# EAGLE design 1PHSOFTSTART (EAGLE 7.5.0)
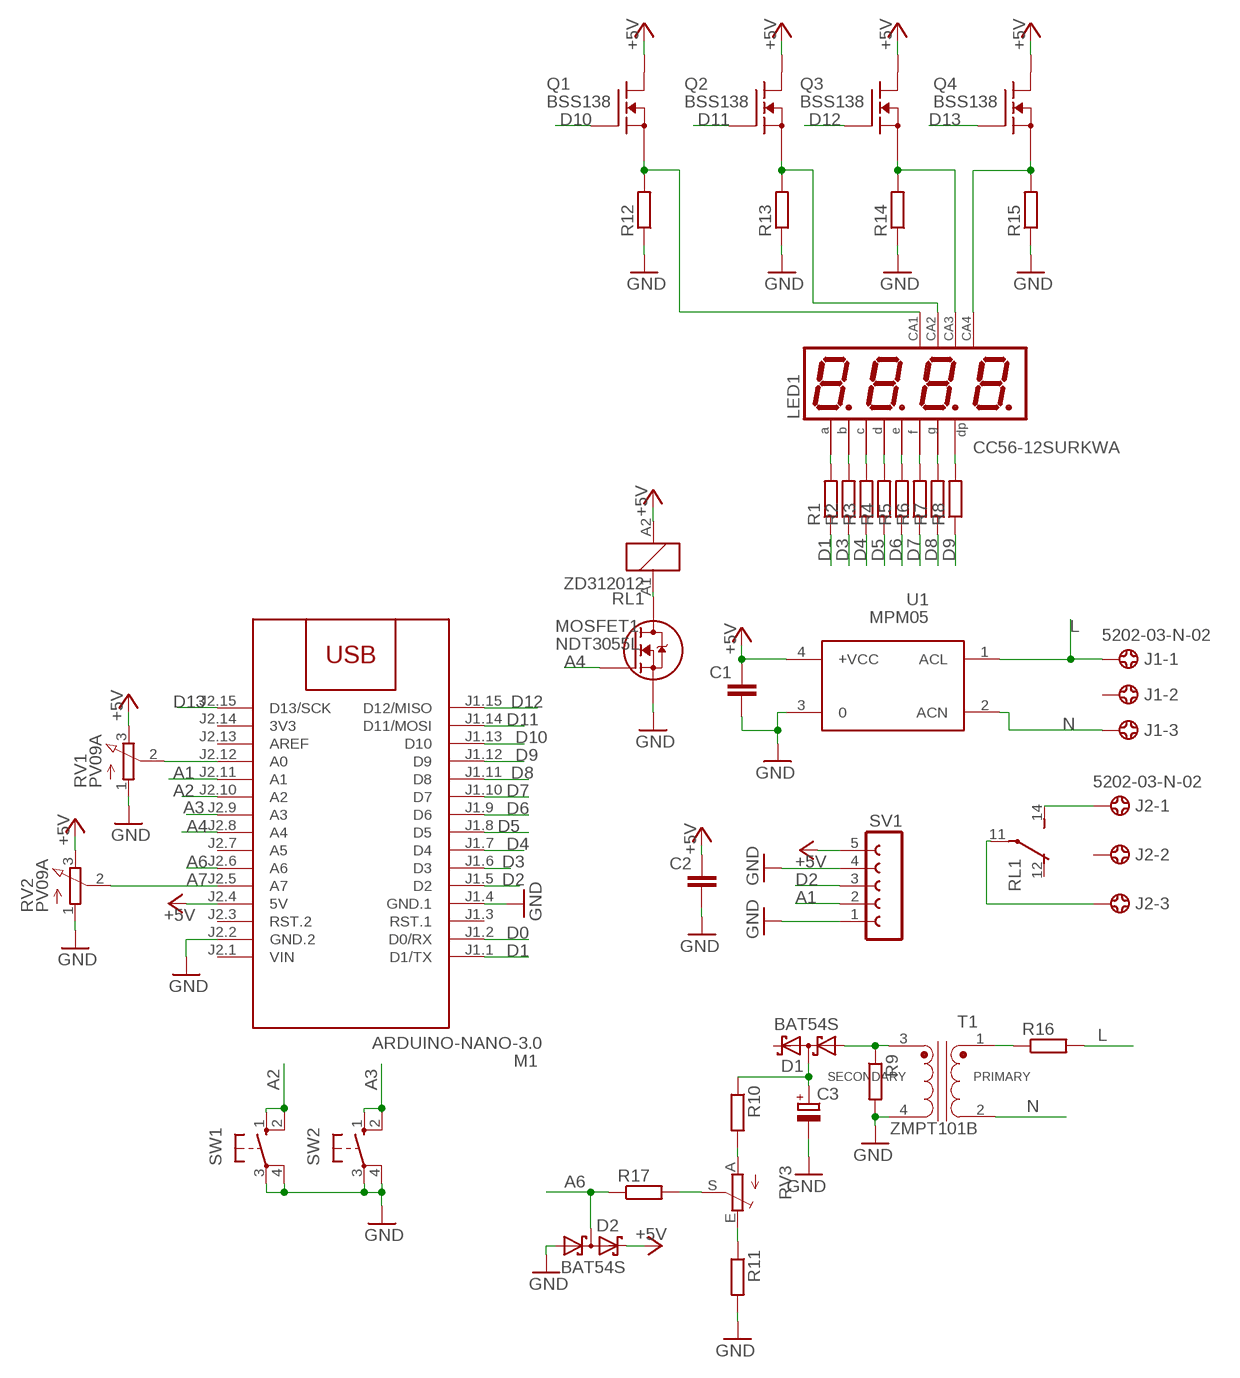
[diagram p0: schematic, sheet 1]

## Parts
C1  C-EUC1206  [C1206]
C2  C-EUC1206  [C1206]
C3  CPOL-EUSMCD  [SMC_D]
D1  BAT54S  [SOT23]
D2  BAT54S  [SOT23]
J1  5202-03-N-02  [5202-03-N-02]
J2  5202-03-N-02  [5202-03-N-02]
LED1  CC56-12SURKWA  CA56-12SURKWA  [CA56-12SURKWA]
M1  ARDUINO-NANO-3.0  [ARDUINO-NANO-3.0]
MOSFET1  NDT3055L  [SOT223-4]
Q1  BSS138  [SOT23]
Q2  BSS138  [SOT23]
Q3  BSS138  [SOT23]
Q4  BSS138  [SOT23]
R1  R-EU_R1206  [R1206]
R2  R-EU_R1206  [R1206]
R3  R-EU_R1206  [R1206]
R4  R-EU_R1206  [R1206]
R5  R-EU_R1206  [R1206]
R6  R-EU_R1206  [R1206]
R7  R-EU_R1206  [R1206]
R8  R-EU_R1206  [R1206]
R9  R-EU_R1206  [R1206]
R10  R-EU_R1206  [R1206]
R11  R-EU_R1206  [R1206]
R12  R-EU_R1206  [R1206]
R13  R-EU_R1206  [R1206]
R14  R-EU_R1206  [R1206]
R15  R-EU_R1206  [R1206]
R16  R-EU_R1206  [R1206]
R17  R-EU_R1206  [R1206]
RL1  ZD312012  [ZD1]
RV1  PV09A  [PTV09]
RV2  PV09A  [PTV09]
RV3  TRIM_EU-B25P  [B25P]
SV1  FE05-1  [FE05-1]
SW1  10-XX  [B3F-10XX]
SW2  10-XX  [B3F-10XX]
T1  ZMPT101B  [XFMR_ZMPT101B]
U1  MPM05  [MPM05]

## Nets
+5V: C1.1 C2.1 D2.2(C2) M1.J2.4(5V) Q1.2(D) Q2.2(D) Q3.2(D) Q4.2(D) RL1.A2 RV1.3(E) RV2.3(E) SV1.5 U1.4(+VCC)
A1: M1.J2.11(A1) SV1.2
A2: M1.J2.10(A2) SW1.1(S) SW1.2(S1)
A3: M1.J2.9(A3) SW2.1(S) SW2.2(S1)
A4: M1.J2.8(A4) MOSFET1.1(G)
A6: D2.3(C1A2) M1.J2.6(A6) R17.1
A7: M1.J2.5(A7) RV2.2(S)
D0: M1.J1.2(D0/RX)
D1: M1.J1.1(D1/TX) R1.1
D2: M1.J1.5(D2) SV1.3
D3: M1.J1.6(D3) R2.1
D4: M1.J1.7(D4) R3.1
D5: M1.J1.8(D5) R4.1
D6: M1.J1.9(D6) R5.1
D7: M1.J1.10(D7) R6.1
D8: M1.J1.11(D8) R7.1
D9: M1.J1.12(D9) R8.1
D10: M1.J1.13(D10) Q1.3(G)
D11: M1.J1.14(D11/MOSI) Q2.3(G)
D12: M1.J1.15(D12/MISO) Q3.3(G)
D13: M1.J2.15(D13/SCK) Q4.3(G)
GND: C1.2 C2.2 C3.- D2.1(A1) M1.J1.4(GND.1) M1.J2.2(GND.2) MOSFET1.3(S) R9.2 R11.2 R12.1 R13.1 R14.1 R15.1 RV1.1(A) RV2.1(A) SV1.1 SV1.4 SW1.3(P) SW1.4(P1) SW2.3(P) SW2.4(P1) T1.4 U1.3
L: J1.1 R16.2 U1.1(ACL)
N: J1.3 T1.2 U1.2(ACN)
N$1: M1.J2.12(A0) RV1.2(S)
N$2: J2.1 RL1.14(2:S)
N$3: J2.3 RL1.11(2:P)
N$4: D1.1(A1) R9.1 T1.3
N$5: R16.1 T1.1
N$6: C3.+ D1.3(C1A2) R10.1
N$7: R10.2 RV3.A
N$8: R17.2 RV3.S
N$9: R11.1 RV3.E
N$10: LED1.11(A) R1.2
N$11: LED1.7(B) R2.2
N$12: MOSFET1.2(D) MOSFET1.4(D) RL1.A1
N$15: LED1.4(C) R3.2
N$16: LED1.2(D) R4.2
N$17: LED1.1(E) R5.2
N$18: LED1.10(F) R6.2
N$19: LED1.5(G) R7.2
N$20: LED1.3(DP) R8.2
N$21: LED1.12(CA) Q1.1(S) R12.2
N$22: LED1.9(CA) Q2.1(S) R13.2
N$23: LED1.8(CA) Q3.1(S) R14.2
N$24: LED1.6(CA4) Q4.1(S) R15.2
Unconnected: D1.2(C2) J1.2 J2.2 M1.J1.3(RST.1) M1.J2.3(RST.2) M1.J2.7(A5) M1.J2.13(AREF) RL1.12(2:O)

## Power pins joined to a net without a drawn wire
3V3: M1.J2.14(3V3)
VIN: M1.J2.1(VIN)

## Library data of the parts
C1 C2 = rcl:C-EU: CAPACITOR, European symbol
C3 = rcl:CPOL-EU: POLARIZED CAPACITOR, European symbol
D1 D2 = diode:BAT54S: Schottky Diodes Pin connection corrected 2011-05-04 Source: Fairchild .. BAT54.pdf
J1 J2 = con-ebyelectro:5202-03-N-02: Barrier Blocks Sreies 5202 Source: http://www.ebyelectro.com/PDF/5202-XX-N-02.pdf; OC_FARNELL: unknown; OC_NEWARK: unknown
LED1 = display-kingbright:CA56-12SURKWA
M1 = diy-modules:ARDUINO-NANO-3.0: Arduino Nano 3.0 and compatible devices More details available here: https://www.arduino.cc/en/Main/ArduinoBoardNano Click here to find device on ebay.com
MOSFET1 = NDT3055L:NDT3055L: Trans MOSFET N-CH 60V 4A 4-Pin(3+Tab) SOT-223 Trans MOSFET N-CH 60V 4A 4-Pin(3+Tab) SOT-223 Check availability; AVAILABILITY: In Stock; CHECK_PRICES: https://www.snapeda.com/parts/NDT3055L/Onsemi/view-part/?ref=eda; DESCRIPTION: Trans MOSFET N-CH 60V 4A 4-Pin(3+Tab) SOT-223 Trans MOSFET N-CH 60V 4A 4-Pin(3+Tab) SOT-223; MF: ON; MP: NDT3055L; PACKAGE: SOT-223-4 Fairchild Semiconductor; PRICE: None; SNAPEDA_LINK: https://www.snapeda.com/parts/NDT3055L/Onsemi/view-part/?ref=snap
Q1-Q4 = transistor-fet:BSS138
R1-R17 = rcl:R-EU_: RESISTOR, European symbol
RL1 = relay:ZD?1*: Power Relay SCHRACK 1 pole 30 A Source: http://www.schrack.com/.. 5848.pdf; OC_FARNELL: unknown; OC_NEWARK: unknown
RV1 RV2 = pot:PV09A
RV3 = pot:TRIM_EU-: POTENTIOMETER
SV1 = con-lsta:FE05-1: FEMALE HEADER; OC_FARNELL: unknown; OC_NEWARK: unknown
SW1 SW2 = switch-omron:10-XX: OMRON SWITCH; MPN: B3F-1000; OC_FARNELL: 176432; OC_NEWARK: 36M3542
T1 = ZMPT101B:ZMPT101B: Check availability; AVAILABILITY: Not in stock; CHECK_PRICES: https://www.snapeda.com/parts/ZMPT101B/Qingxian+Zeming+Langxi+Electronic/view-part/?ref=eda; DESCRIPTION: Current-type Voltage Transformer; MF: Qingxian Zeming Langxi Electronic; MP: ZMPT101B; PACKAGE: None; PRICE: None; SNAPEDA_LINK: https://www.snapeda.com/parts/ZMPT101B/Qingxian+Zeming+Langxi+Electronic/view-part/?ref=snap
U1 = acdc:MPM05: AC DC Converter 5W

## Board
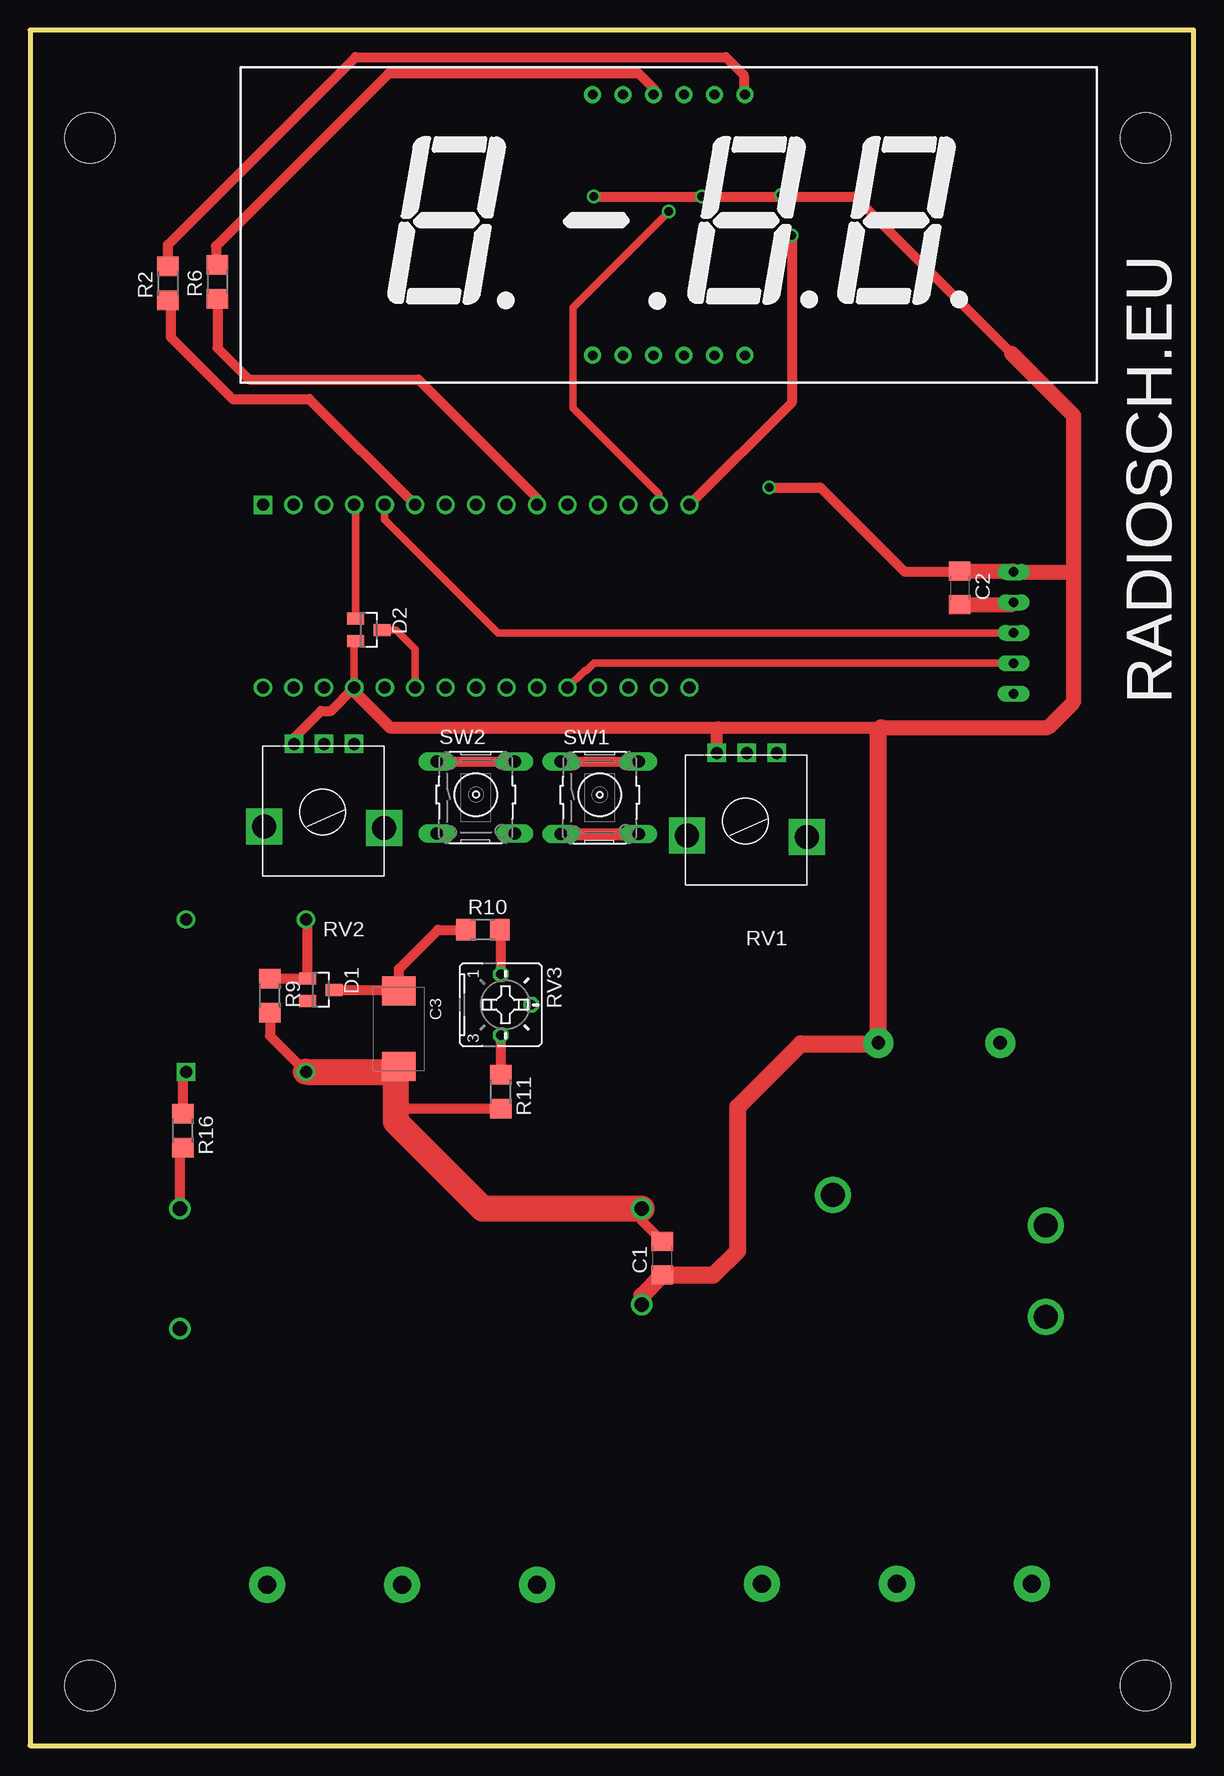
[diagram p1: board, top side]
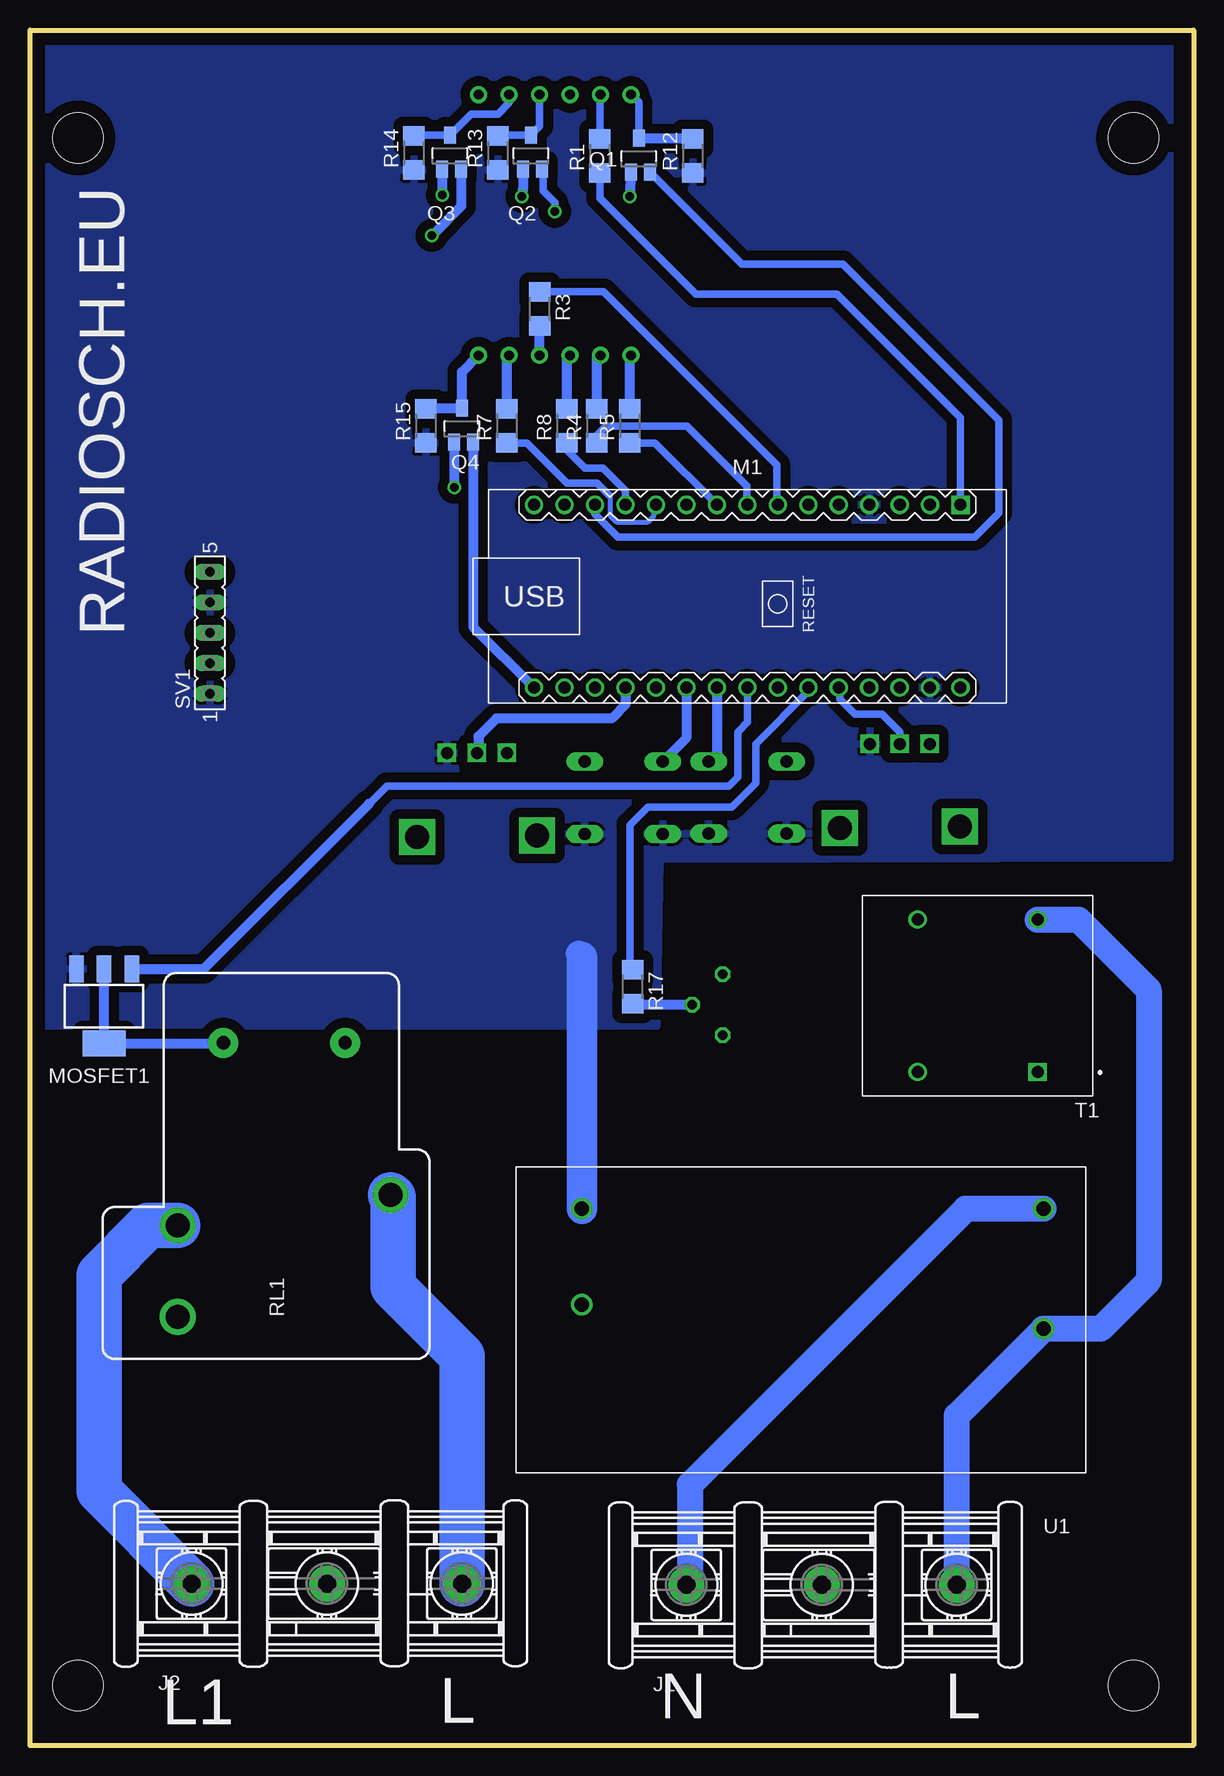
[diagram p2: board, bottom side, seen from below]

Size 97 x 143 mm. Coordinates in mm from the lower left corner, seen from the top.
Outline: 0,0 97,0 97,143 0,143 0,0
Copper layers (1*16): Top 0.035mm / dielectric 1.5mm / Bottom 0.035mm
Design rules "default": minimum track width 10mil, minimum drill 24mil, track to track 8mil, track to pad 8mil, pad to pad 8mil, via to via 8mil, smd to smd 8mil, copper to edge 40mil, drill to drill 8mil, minimum pad ring 10mil, minimum via ring 8mil, stop-mask expansion 4mil, vias tented up to drill 0mil, thermal gap 10mil
Holes 4.2 mm at 5,134 5,5 93,134 93,5

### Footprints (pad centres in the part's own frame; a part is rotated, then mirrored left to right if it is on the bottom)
C1206 = smd 1.6 x 1.8: 1 -1.4,0; 2 1.4,0
SMC_D = smd 2.4 x 2.8: + -3.15,0; - 3.15,0
SOT23 = smd 1 x 1.4: 1 -0.95,-1.1; 2 0.95,-1.1; 3 0,1.1
5202-03-N-02 = drill 1.5 pad 3: 1 -9.29,0; 2 2,0; 3 13.25,0
CA56-12SURKWA = drill 0.8 pad 1.422: 1 10.65,-7.12; 2 13.19,-7.12; 3 15.73,-7.12; 4 18.27,-7.12; 5 20.81,-7.12; 6 23.35,-7.12; 7 23.35,14.62; 8 20.81,14.62; 9 18.27,14.62; 10 15.73,14.62; 11 13.19,14.62; 12 10.65,14.62
ARDUINO-NANO-3.0 = drill 1 square: J1.1 17.78,7.62 | drill 1: J1.2 15.24,7.62; J1.3 12.7,7.62; J1.4 10.16,7.62; J1.5 7.62,7.62; J1.6 5.08,7.62; J1.7 2.54,7.62; J1.8 0,7.62; J1.9 -2.54,7.62; J1.10 -5.08,7.62; J1.11 -7.62,7.62; J1.12 -10.16,7.62; J1.13 -12.7,7.62; J1.14 -15.24,7.62; J1.15 -17.78,7.62; J2.1 17.78,-7.62; J2.2 15.24,-7.62; J2.3 12.7,-7.62; J2.4 10.16,-7.62; J2.5 7.62,-7.62; J2.6 5.08,-7.62; J2.7 2.54,-7.62; J2.8 0,-7.62; J2.9 -2.54,-7.62; J2.10 -5.08,-7.62; J2.11 -7.62,-7.62; J2.12 -10.16,-7.62; J2.13 -12.7,-7.62; J2.14 -15.24,-7.62; J2.15 -17.78,-7.62
SOT223-4 = smd 1.219 x 2.235: 1 -2.24,-3.091; 2 0.071,-3.091; 3 2.383,-3.091 | smd 3.6 x 2.2: 4 0.071,3.107
SOT23' = smd 1 x 1.4: 1 0,1.735; 2 -0.632,-1.1; 3 0.95,-1.1
R1206 = smd 1.6 x 1.803: 1 -1.422,0; 2 1.422,0
ZD1 = drill 2 pad 2.5: 11 -2.54,-8.88; 12 -12.7,8.88; 14 -5.08,8.88 | drill 1.1 pad 2.5: A1 10.16,5.08; A2 10.16,-5.08
PTV09 = drill 1 square: 1 -2.5,0; 2 0,0; 3 2.5,0 | drill 2 square: P$4 -5,7; P$5 5,6.9
B25P = drill 0.813 octagon: A -2.54,0; E 2.54,0; S 0,2.54
FE05-1 = drill 0.813 long: 1 -5.08,0; 2 -2.54,0; 3 0,0; 4 2.54,0; 5 5.08,0
B3F-10XX = drill 1.016 long: 1 -3.251,2.761; 2 3.251,2.761; 3 -3.251,-3.261; 4 3.251,-3.261
XFMR_ZMPT101B = drill 1 square: 1 -5,6.35 | drill 1: 2 -5,-6.35; 3 5,-6.35; 4 5,6.35
MPM05 = drill 1.2: 1 3.5,-22; 2 3.5,-12; 3 42,-22; 4 42,-14

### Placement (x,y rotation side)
C1  52.72,40.62 90 top
C2  77.5,96.5 270 top
C3  30.75,59.75 270 top
D1  24.25,63 270 top
D2  28.25,93 270 top
J1  33,13.39 0 bottom
J2  74.25,13.5 0 bottom
LED1  36.25,123 0 top
M1  37.2,95.8 0 bottom
MOSFET1  90.75,61.62 180 bottom
Q1  BSS138  [SOT23']  46.25,132.25 0 bottom
Q2  BSS138  [SOT23']  55.25,132.5 0 bottom
Q3  BSS138  [SOT23']  62,132.5 0 bottom
Q4  BSS138  [SOT23']  61,109.75 0 bottom
R1  49.5,132.5 90 bottom
R2  11.5,121.88 90 top
R3  54.5,119.75 270 bottom
R4  49.75,110 90 bottom
R5  47,110 90 bottom
R6  15.62,122 90 top
R7  57.25,110 90 bottom
R8  52.25,110 90 bottom
R9  20,62.5 270 top
R10  37.75,68 0 top
R11  39.25,54.5 270 top
R12  41.75,132.5 90 bottom
R13  58,132.75 90 bottom
R14  65,132.75 90 bottom
R15  64,110 90 bottom
R16  12.75,51.25 270 top
R17  46.75,63.25 270 bottom
RL1  75.8,48.42 90 bottom
RV1  59.75,82.75 180 top
RV2  24.5,83.5 180 top
RV3  39.25,61.75 270 top
SV1  82,92.75 90 bottom
SW1  47.5,79.25 0 top
SW2  37.17,79.27 0 top
T1  18,62.5 180 bottom
U1  9,22.75 180 bottom

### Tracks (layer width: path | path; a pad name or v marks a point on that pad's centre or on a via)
+5V  (via drill 0.7)
  Top 0.61: M1.J2.4 27.04,91.94 D2.2
  Top 0.813: v47,129.12 v56,129.12 62.5,129.12 | 62.5,129.12 v62.62,129.25 | 62.5,129.12 68.75,129.12 81.81,116.06 82,115.88 | v61.62,104.88 65.88,104.88 72.88,97.88 77.47,97.88 C2.1 | RV2.3 22,84 24.25,86.25 25.11,86.25 M1.J2.4
  Top 1.016: M1.J2.4 27.04,87.84 30,84.88 57.38,84.88 | 57.38,84.88 71,84.88 | RV1.3 57.25,84.75 57.38,84.88
  Top 1.27: 70.97,84.84 71,84.88 84.88,84.88 87,87 87,97.75 | 87,97.75 87,110.88 81.81,116.06 | 87,97.75 86.92,97.83 SV1.5 81.93,97.9 C2.1
  Top 1.422: U1.4 51,37.5 C1.1 56.97,39.22 59,41.25 59,53.25 64.25,58.5 70.64,58.5 RL1.A2 70.72,84.59 70.97,84.84
  Bottom 0.61: 61.5,104.75 v61.62,104.88
  Bottom 0.813: v47,129.12 Q1.2 | Q2.2 55.88,130.01 v56,129.12 | Q3.2 62.63,130.12 v62.62,129.25 | Q4.2 61.63,104.88 v61.62,104.88
A1
  Top 0.61: M1.J2.11 46.27,89.62 46.38,89.62 47,90.25 81.96,90.25 SV1.2
A2
  Top 0.813: SW1.1 SW1.2
  Bottom 0.813: M1.J2.10 42.28,83.98 SW1.1
A3
  Top 0.813: SW2.1 SW2.2
  Bottom 0.813: M1.J2.9 39.74,82.71 SW2.2
A4
  Bottom 0.61: M1.J2.8 37.2,85.3 38,84.5 38,80.75 38.75,80 67.25,80 68.75,78.5
  Bottom 0.813: MOSFET1.1 82.52,64.73 68.75,78.5
A6
  Top 0.61: M1.J2.6 32.12,91.38 30.5,93 D2.3
  Bottom 0.61: M1.J2.6 32.12,87.88 36.5,83.5 36.5,80.25 38.5,78.25 45.5,78.25 47,76.75 47,64.92 R17.1
A7
  Bottom 0.61: RV2.2 24.5,84.5 26,86 28.25,86 29.5,87.25 29.5,88.1 M1.J2.5
D1
  Bottom 0.61: M1.J1.1 19.42,110.67 29.75,121 41.5,121 49.5,129 R1.1
D2
  Top 0.61: M1.J1.5 29.58,102.17 39,92.75 SV1.3
D3
  Top 0.813: R2.1 11.75,120.2 11.75,117.38 16.88,112.25 23.29,112.25 M1.J1.6
D4
  Bottom 0.61: R3.1 49.17,121.17 34.75,106.75 34.75,103.51 M1.J1.7
D5
  Bottom 0.61: M1.J1.8 37.25,103.47 37.25,105 42.25,110 49,110 49.75,109.25 R4.1
D6
  Bottom 0.61: R5.1 44.9,108.58 M1.J1.9
D7
  Top 0.813: R6.1 15.62,116.5 18.25,113.88 32.38,113.88 42.25,104 42.25,103.45 M1.J1.10
D8
  Bottom 0.406: M1.J1.11 45,103.24 45,102.5 45.5,102 48.12,102 48.62,102.5 48.62,104.12 48.75,104.25
  Bottom 0.61: R7.1 55.58,108.58 52.25,105.25 49.75,105.25 48.75,104.25
D9
  Bottom 0.61: M1.J1.12 47.36,104.61 49.25,106.5 50.75,106.5 52.25,108 R8.1
D10
  Bottom 0.61: M1.J1.13 49.9,102.65 48,100.75 18.25,100.75 16.25,102.75 16.25,110.5 29.25,123.5 37.65,123.5 Q1.3
D11  (via drill 0.7)
  Top 0.61: M1.J1.14 52.44,104.31 45.25,111.5 45.25,119.88 v53.25,127.88
  Bottom 0.61: v53.25,127.88 53.25,128.62 54.25,129.62 54.25,131.35 Q2.3
D12  (via drill 0.7)
  Top 0.813: v63.5,125.88 63.5,111.94 M1.J1.15
  Bottom 0.813: Q3.3 61.05,128.32 v63.5,125.88
D13
  Bottom 0.813: Q4.3 60.05,93.25 M1.J2.15
GND
  Top 0.61: D2.1 27.15,103.31 M1.J1.4
  Top 0.813: R9.2 20,59.15 T1.4 | R11.2 30.58,53.08 30.5,53 | U1.3 51,43.74 C1.2
  Top 1.016: SW1.3 SW1.4
  Top 1.27: C2.2 81.81,95.1 SV1.4
  Top 2.184: U1.3 37.75,44.75 30.5,52 30.5,53 30.5,56.35 C3.- 30.3,56.15 T1.4
  Bottom 2.184: 51,65.75 51.25,66
  Bottom 2.54: U1.3 51,65.75
  pour Bottom (isolate 0.813): 2,142 96,142 95.75,60 44.75,60 44.5,73.88 2,74
L
  Top 0.813: U1.1 12.5,49.58 R16.2
  Bottom 2.184: U1.1 19,44.75 42,21.75 42,13.68 J1.1
N
  Bottom 2.184: J1.3 19.75,27.5 U1.2 7.75,34.75 3.75,38.75 3.75,63 9.6,68.85 T1.2
N$1
  Bottom 0.813: M1.J2.12 47.36,86.77 48.5,85.62 58.12,85.62 59.62,84.12 59.62,82.88 RV1.2
N$2
  Bottom 3.81: RL1.14 87.16,43.34 91.25,39.25 91.25,21.21 J2.1
N$3
  Bottom 3.81: J2.3 61,32.5 66.75,38.25 66.75,45.71 RL1.11
N$4
  Top 0.813: T1.3 23.15,68.7 D1.1 23.12,63.92 R9.1
N$5
  Top 0.813: R16.1 12.75,55.9 T1.1
N$6
  Top 0.813: D1.3 30.65,63 C3.+ 30.75,64.75 34,68 R10.1
N$7
  Top 0.813: RV3.A 39.25,67.92 R10.2
N$8
  Bottom 0.813: RV3.S 46.67,61.75 R17.2
N$9
  Top 0.813: R11.1 RV3.E
N$10
  Bottom 0.61: R1.2 49.5,137.56 LED1.11
N$11
  Top 0.813: R2.2 11.5,125.12 27.12,140.75 58,140.75 59.5,139.25 59.5,137.72 LED1.7
N$12
  Bottom 0.813: MOSFET1.2 MOSFET1.4 80.94,58.52 RL1.A1
N$15
  Bottom 0.813: LED1.4 54.52,118.31 R3.2
N$16
  Bottom 0.813: R4.2 49.75,115.57 LED1.2
N$17
  Bottom 0.813: R5.2 47,115.78 LED1.1
N$18
  Top 0.813: LED1.10 51.98,138.14 50.75,139.38 29.88,139.38 15.5,125 15.5,123.55 R6.2
N$19
  Bottom 0.813: R7.2 57.25,115.69 LED1.5
N$20
  Bottom 0.813: R8.2 52.25,115.61 LED1.3
N$21
  Bottom 0.61: Q1.1 46.25,136.97 LED1.12
  Bottom 0.813: R12.2 46.19,133.92 Q1.1
N$22
  Bottom 0.61: LED1.9 54.52,134.97 Q2.1 57.94,134.24 R13.2
N$23
  Bottom 0.61: LED1.8 57.06,136.94 58,136 60.23,136 Q3.1 64.94,134.24 R14.2
N$24
  Bottom 0.61: 61.06,111.42 Q4.1
  Bottom 0.813: 61.06,111.42 R15.2 | Q4.1 61,114.48 LED1.6

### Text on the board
tPlace: RADIOSCH.EU
bPlace: RADIOSCH.EU | L | N | L | L1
